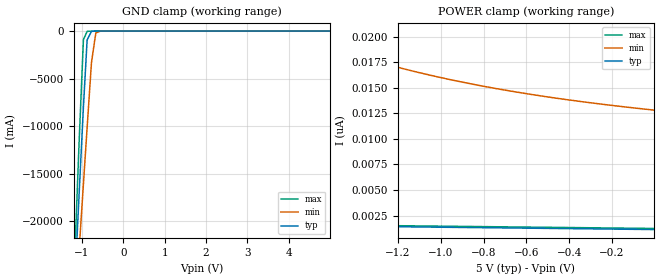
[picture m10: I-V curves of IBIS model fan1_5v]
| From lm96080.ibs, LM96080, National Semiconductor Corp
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[Model] fan1_5v
Model_type Input
Vinh = 3.5V
Vinl = 1.5V
C_comp   3.02pF   2.81pF   3.44pF
[Voltage Range]   5.0V   4.5V   5.5V
[Temperature Range]   25.0   125.0   -40.0
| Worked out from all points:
|   GND clamp passes 1 mA (typ) near -0.60 V on its own axis
[GND Clamp]
-5V       -363A      -283.2A    -452.2A
-1.175V   -26.61A    -30.2A     -23.67A
-1.07V    -17.23A    -23.11A    -11.79A
-965mV    -7.991A    -16.08A    -906mA
-875mV    -930.4mA   -10.14A    -30.97mA
-770mV    -30.76mA   -3.312A    -3.487mA
-665mV    -2.472mA   -195.5mA   -254.8uA
-560mV    -172.6uA   -14.29mA   -9.002uA
-470mV    -13.52uA   -1.763mA   -315.8nA
4.99V     1.129nA    0A         1.123nA
[POWER Clamp]
-5V       2.432nA    133.4nA    2.363nA
-3.575V   1.996nA    55.58nA    2.042nA
-1.715V   1.527nA    20.53nA    1.623nA
-1.61V    1.502nA    19.68nA    1.6nA
-1.505V   1.478nA    18.91nA    1.576nA
-1.355V   1.443nA    17.91nA    1.542nA
-1.16V    1.397nA    16.79nA    1.498nA
-950mV    1.349nA    15.78nA    1.451nA
-755mV    1.304nA    14.98nA    1.407nA
-500mV    1.245nA    14.11nA    1.35nA
-245mV    1.187nA    13.39nA    1.293nA
-5mV      1.132nA    12.82nA    1.239nA
